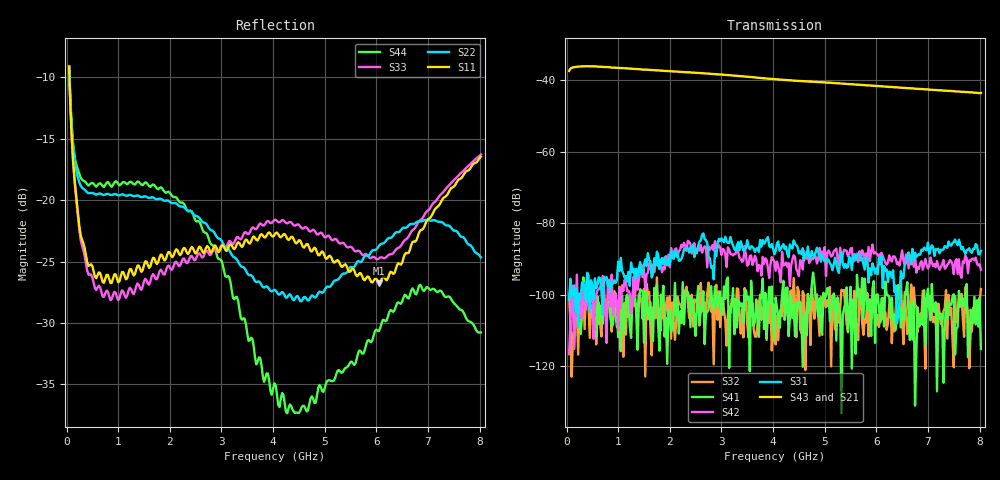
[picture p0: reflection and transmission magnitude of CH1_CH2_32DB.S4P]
!Agilent Technologies,E5071C,MY46316741,A.11.02
!Date: Thu May 28 14:28:03 2026
!Data & Calibration Information:
!1:CH1 INPUT 2:CH1 OUTPUT 3:CH2 INPUT 4:CH2 OUTPUT
!Freq	S11:SOLT4(ON)	S12:SOLT4(ON)	S13:SOLT4(ON)	S14:SOLT4(ON)
!	S21:SOLT4(ON)	S22:SOLT4(ON)	S23:SOLT4(ON)	S24:SOLT4(ON)
!	S31:SOLT4(ON)	S32:SOLT4(ON)	S33:SOLT4(ON)	S34:SOLT4(ON)
!	S41:SOLT4(ON)	S42:SOLT4(ON)	S43:SOLT4(ON)	S44:SOLT4(ON)
!PortZ  Port1:50+j0  Port2:50+j0  Port3:50+j0  Port4:50+j0
!Above PortZ is port z conversion or system Z0 setting when saving the data.
!When reading, reference impedance value at option line is always used.
# Hz S dB R 50
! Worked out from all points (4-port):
!   320 points, 50 MHz to 8.025 GHz, reference 50 ohm
!   strongest paths, dB at 50 MHz, 2.05 GHz, 4.05 GHz, 6.05 GHz, 8.025 GHz:
!     S43: -37.4, -37.5, -39.7, -41.6, -43.6
!     S21: -37.4, -37.6, -39.8, -41.7, -43.5
!     S31: -101.6, -89.5, -87.8, -89.8, -87.7
!     S42: -116.7, -88.9, -93.3, -89.5, -93.0
!     S41: -100.3, -109.0, -100.8, -103.3, -115.2
!     S32: -100.2, -102.2, -113.9, -109.0, -98.4
!   lowest |S11| = -26.8 dB at 6.05 GHz (marker M1), VSWR 1.10, Z = 47.1 - j3.38 ohm
!   |S11| at or under -10 dB: 56.68 MHz to end of sweep
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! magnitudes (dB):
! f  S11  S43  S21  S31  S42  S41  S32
! 50 MHz  -9.1  -37.4  -37.4  -101.6  -116.7  -100.3  -100.2
! 275 MHz  -22.9  -36.1  -36.2  -101.2  -101.8  -111.0  -110.0
! 700 MHz  -26.7  -36.3  -36.4  -105.4  -94.8  -108.1  -103.7
! 2.425 GHz  -23.8  -37.8  -37.9  -86.9  -88.5  -101.1  -100.0
! 4.275 GHz  -23.2  -40.0  -40.0  -88.5  -92.1  -98.0  -104.4
! 6.05 GHz  -26.8  -41.6  -41.7  -89.8  -89.5  -103.3  -109.0
! 8.025 GHz  -16.5  -43.6  -43.5  -87.7  -93.0  -115.2  -98.4
